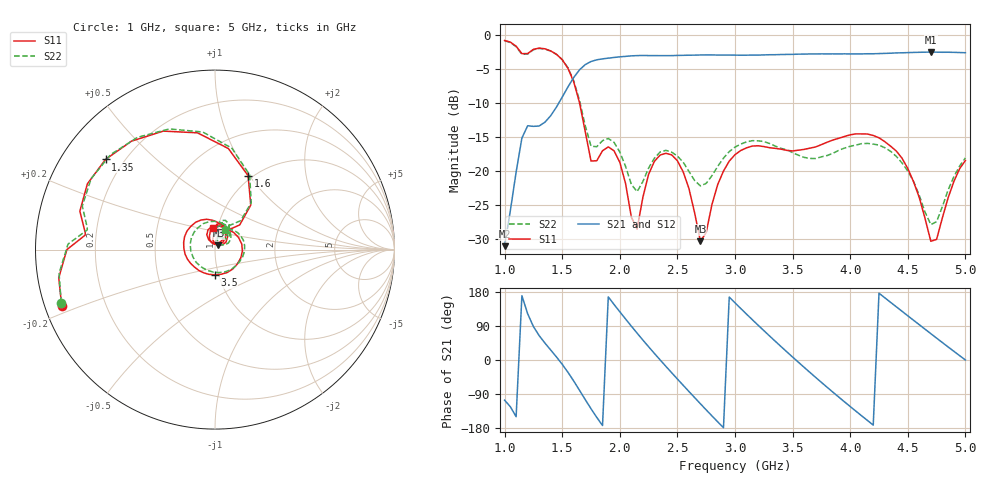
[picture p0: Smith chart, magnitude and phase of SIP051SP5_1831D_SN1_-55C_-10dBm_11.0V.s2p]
# GHz  S  dB  R  50
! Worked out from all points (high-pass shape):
!   81 points, 1 GHz to 5 GHz, reference 50 ohm
!   highest |S21| = -2.53 dB at 4.7 GHz (marker M1); lowest = -31.1 dB at 1 GHz (marker M2)
!   |S21| within 3 dB of the highest: 1.633 GHz to end of sweep
!   lowest |S11| = -30.4 dB at 2.7 GHz (marker M3), VSWR 1.06, Z = 51.9 + j2.46 ohm
!   |S11| at or under -10 dB: 1.651 GHz to end of sweep
!   |S22| runs from -27.9 to -0.9 dB; largest |S21 - S12| = 0.0023
!   S11 on the Smith chart (normalised r, x): 1 GHz: 0.05, -0.18; 1.35 GHz: 0.13, +0.35; 1.6 GHz: 0.95, +0.99; 3.5 GHz: 0.96, -0.27; 5 GHz: 0.95, +0.23
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1  -0.82 -159.7  -31.07 -106.0  -31.04 -106.1  -0.85 -160.9
1.15  -2.76 173.6  -15.18 169.7  -15.18 169.7  -2.85 171.2
1.35  -2.04 140.5  -12.84 44.7  -12.83 44.5  -2.09 137.7
1.5  -3.64 98.5  -9.15 -11.3  -9.14 -11.4  -3.63 95.9
1.6  -6.91 65.9  -6.26 -55.4  -6.25 -55.5  -6.76 65.1
1.7  -14.23 45.0  -4.37 -104.5  -4.37 -104.5  -13.35 48.4
1.85  -17.03 86.6  -3.52 -173.0  -3.51 -173.0  -15.55 76.7
2.05  -21.85 50.3  -3.16 108.2  -3.16 108.2  -19.33 49.8
2.15  -28.55 104.3  -3.04 70.9  -3.05 70.9  -23.05 73.7
2.35  -17.67 96.8  -3.05 0.3  -3.05 0.3  -17.22 77.9
2.55  -20.14 44.8  -3.00 -66.7  -3.00 -66.6  -18.71 44.9
2.7  -30.37 51.3  -2.95 -115.6  -2.95 -115.6  -22.20 53.1
2.85  -22.00 95.6  -2.96 -163.2  -2.96 -163.1  -19.34 65.7
3  -17.61 56.9  -2.98 150.8  -2.97 150.8  -16.51 46.1
3.25  -16.42 -17.7  -2.94 77.7  -2.95 77.6  -15.69 -3.4
3.5  -17.06 -90.9  -2.86 7.8  -2.86 7.8  -17.32 -65.2
3.7  -16.48 -139.5  -2.81 -45.9  -2.80 -45.9  -18.18 -128.8
3.95  -14.94 167.1  -2.79 -110.3  -2.79 -110.2  -16.65 153.1
4.15  -14.58 125.3  -2.77 -159.5  -2.77 -159.6  -15.96 101.2
4.35  -16.36 83.9  -2.69 152.3  -2.71 152.4  -17.11 58.1
4.7  -30.35 66.0  -2.53 69.5  -2.54 69.5  -27.90 45.3
5  -18.47 96.3  -2.62 0.1  -2.62 0.1  -18.09 63.0
